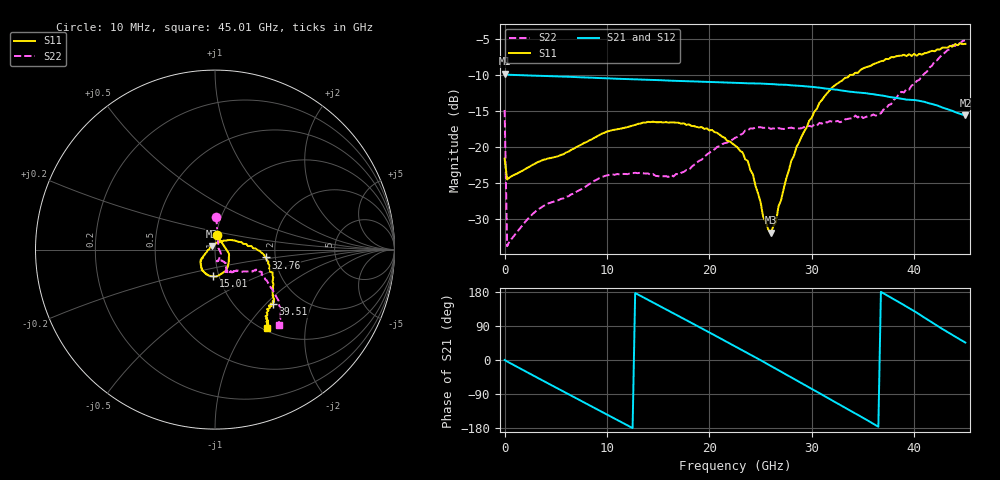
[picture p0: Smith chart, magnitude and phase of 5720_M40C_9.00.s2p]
! Device:  ADRF5720
! Description: 0.5dB LSB GaAs MMIC 6-bit Digital Attenuator
! Frequency:  0.000009 -  40 GHz
! Ports:
!	RF1	= Port 1
!	RF2	= Port 2
! Vdd:  3.3 Volt
! Vss:  -3.3 Volt
! Control:  0/3.3 Volt
! State:  9.00 dB attenuation
! Data:  The device was measured using G-S-G Probes on a matrix board.
!  Data was collected using an calibrated 4 port network analyzer.
!  The reference plane for this measurement is at the launchers.
! Note:  Analog Devices supplies this data as a sample of measured data
!  for this product.  Your particular data for this product may vary.
!  Data was taken at -40 degrees C.
!  Analog Devices reserves the right to change this data at anytime.
# GHZ S DB R 45.0
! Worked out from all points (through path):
!   181 points, 10 MHz to 45.01 GHz, reference 45 ohm
!   highest |S21| = -9.74 dB at 10 MHz (marker M1); lowest = -15.6 dB at 45.01 GHz (marker M2)
!   group delay of S21, straight-line fit = 41.2 ps
!   lowest |S11| = -31.9 dB at 26.01 GHz (marker M3), VSWR 1.05, Z = 43.5 + j1.73 ohm
!   |S11| at or under -10 dB: start of sweep to 33.7 GHz
!   |S22| runs from -33.8 to -5.1 dB; largest |S21 - S12| = 0.0013
!   S11 on the Smith chart (normalised r, x): 10 MHz: 1.00, +0.17; 15.01 GHz: 0.94, -0.29; 32.76 GHz: 1.77, -0.17; 39.51 GHz: 1.46, -1.10; 45.01 GHz: 1.04, -1.26
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0.01  -21.58 83.7  -9.74 -0.1  -9.76 -0.1  -14.81 87.7
0.26  -24.48 6.8  -9.90 -4.0  -9.92 -4.0  -33.76 19.9
2.26  -22.85 -9.3  -10.01 -33.0  -10.03 -33.1  -29.99 -21.4
4.26  -21.55 -19.7  -10.10 -61.8  -10.12 -61.8  -27.82 -36.3
7.76  -19.41 -45.1  -10.28 -111.9  -10.30 -111.9  -25.58 -62.3
11.51  -17.36 -69.6  -10.49 -165.4  -10.51 -165.5  -23.71 -76.8
15.01  -16.52 -93.4  -10.66 144.6  -10.68 144.5  -24.02 -76.5
15.26  -16.50 -95.1  -10.67 140.9  -10.69 140.9  -24.06 -76.0
19.01  -17.25 -118.0  -10.87 87.0  -10.89 86.9  -21.88 -55.1
22.76  -20.04 -143.9  -11.05 32.6  -11.07 32.5  -18.53 -58.0
23.76  -21.90 -149.1  -11.10 18.0  -11.12 17.9  -17.65 -60.6
25.26  -29.70 178.4  -11.15 -4.3  -11.17 -4.4  -17.30 -62.6
26.01  -31.88 128.9  -11.21 -15.5  -11.23 -15.6  -17.46 -63.4
26.51  -30.41 87.9  -11.25 -23.1  -11.27 -23.2  -17.49 -64.8
28.01  -21.87 38.5  -11.38 -45.6  -11.40 -45.8  -17.26 -64.6
30.26  -15.05 10.2  -11.63 -80.1  -11.66 -80.3  -16.83 -61.1
32.76  -10.90 -8.8  -12.07 -118.3  -12.09 -118.5  -16.52 -55.2
35.26  -8.88 -25.5  -12.47 -156.3  -12.50 -156.5  -15.79 -47.3
37.76  -7.46 -39.6  -13.04 164.3  -13.06 164.1  -14.00 -37.3
39.51  -7.06 -43.2  -13.39 137.3  -13.42 137.2  -11.98 -26.3
42.01  -6.64 -52.8  -14.09 94.7  -14.11 94.5  -8.03 -35.2
45.01  -5.61 -56.4  -15.55 46.0  -15.59 45.9  -5.14 -49.7
